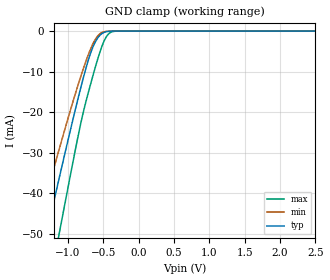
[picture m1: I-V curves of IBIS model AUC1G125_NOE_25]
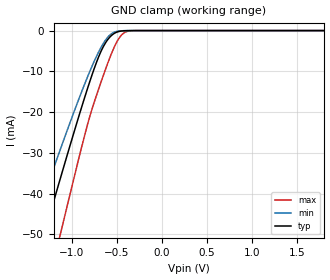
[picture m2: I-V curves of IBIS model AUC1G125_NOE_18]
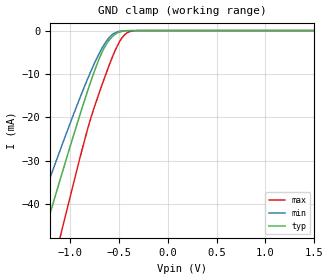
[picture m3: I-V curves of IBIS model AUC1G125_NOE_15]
| TEXAS INSTRUMENTS INCORPORATED
| Standard Linear and Logic Group
| IBIS Model of SN74AUC1G125
| Single Bus Buffer Gate with 3-State Output
| This file contains package information for the following:
|  SOT 5-pin (DBV) package as [Component] AUC1G125_DBV
|  SOT 5-pin (DCK) package as [Component] AUC1G125_DCK
|  DSBGA 5-pin (YEA) package as [Component] AUC1G125_YEA
|  DSBGA 5-pin (YZA) package as [Component] AUC1G125_YZA
|  DSBGA 5-pin (YEP) package as [Component] AUC1G125_YEP
|  DSBGA 5-pin (YZP) package as [Component] AUC1G125_YZP
| This device can be powered at the following Vccs:
|  2.5 volt Vcc
|  1.8 volt Vcc
|  1.5 volt Vcc
|  1.2 volt Vcc
|  0.8 volt Vcc
| This file provides unique models under the [Model Selector] for each Vcc.
| For operation at a specific Vcc, select the appropriate model after each
| [Model Selector] keyword.
[IBIS Ver]   3.2
[Comment char]  |_char
[File Name]   sn74auc1g125.ibs
[File Rev]   1.3 | x_die
[Date]   July 27, 2004
[Source]   Data created from TI-SPICE simulations at TI-SLL.
[Notes]   The following is an IBIS list for the SN74AUC1G125.
   Please contact sllibis@ti.com with questions and
   comments concerning SLL IBIS models.
   - FILE REV HISTORY
   - 1.3 YEP and YZP packages added on 07/27/04
   - The SN74AUC1G125 has output feedback control circuitry.
   This will cause some non-monotonicity warnings.
   - The SN74AUC1G125 inputs has no power clamp diode.
   Therefore, the input power clamp data are not included.
   - The SN74AUC1G125 outputs has no power clamp diode.
   Therefore, the output power clamp data are not included.
   - End point warning due to AC and DC mismatch.
[Disclaimer] Property of Texas Instruments Incorporated.  Unauthorized
   reproduction and/or distribution is strictly prohibited.
   This product is protected under copyright law.
   Created  2002, (C) Copyright  2002, Texas Instruments
   Incorporated, All Rights Reserved
   UNLESS THERE IS A SIGNED, WRITTEN AGREEMENT TO THE
   CONTRARY, TEXAS INSTRUMENTS (TI) IS PROVIDING THE IBIS
   MODELS  AND WITHOUT ANY WARRANTY, EXPRESSED OR
   IMPLIED.  TI assumes no liability for:
   1) the accuracy of the IBIS models provided to your
   company;
   2) the proper functioning of these IBIS Models in your
   design or for any resulting applications; or
   3) infringement of patents, copyrights or intellectual
   property rights resulting from your use of these IBIS
   models.
   TI provides IBIS Models as a service to our customers.
   You and your company shall not distribute, sell or give
   these models to anyone else without prior written
   permission from TI.
   TI reserves the right to make changes to our products or
   to discontinue any semiconductor product or service
   without notice, and advises our customers to obtain the
   latest version of relevant information to verify, before
   placing orders, that the information being relied on is
   current.
   Please be aware that your receipt and use of the IBIS
   information provided shall serve as acceptance of these
   terms and conditions.  If you do not accept these terms,
   you should return or destroy the IBIS models and any
   other accompanying information immediately.
| Component AUC1G125_DBV 5-pin SOT
[Component]   AUC1G125_DBV
[Manufacturer]   Texas Instruments, Inc.
[Package]
|   typ   min   max
R_pkg   2.500e-02   2.100e-02   2.900e-02
L_pkg   1.529e-09   1.312e-09   1.906e-09
C_pkg   1.560e-13   1.100e-13   2.400e-13
[Pin]   signal_name   model_name   R_pin   L_pin   C_pin
1   NOE   AUC1G125_NOE   2.100e-02   1.511e-09   1.440e-13
2   A   AUC1G125_IN   2.300e-02   1.312e-09   1.380e-13
3   GND   GND   2.900e-02   1.906e-09   2.400e-13
4   Y   AUC1G125_OUT   2.600e-02   1.541e-09   1.500e-13
5   VCC   POWER   2.500e-02   1.374e-09   1.100e-13
| Component AUC1G125_DCK 5-pin SOT
[Component]   AUC1G125_DCK
[Manufacturer]   Texas Instruments, Inc.
[Package]
|   typ   min   max
R_pkg   2.000e-02   1.700e-02   2.500e-02
L_pkg   9.980e-10   8.810e-10   1.069e-09
C_pkg   1.460e-13   1.180e-13   2.050e-13
[Pin]   signal_name   model_name   R_pin   L_pin   C_pin
1   NOE   AUC1G125_NOE   1.900e-02   1.069e-09   1.620e-13
2   A   AUC1G125_IN   1.800e-02   8.810e-10   1.210e-13
3   GND   GND   1.700e-02   1.031e-09   2.050e-13
4   Y   AUC1G125_OUT   2.000e-02   9.600e-10   1.240e-13
5   VCC   POWER   2.500e-02   1.049e-09   1.180e-13
| Component AUC1G125_YEA 5-pin NanoStar WCSP
[Component]   AUC1G125_YEA
[Manufacturer]   Texas Instruments, Inc.
[Package]
|   typ   min   max
R_pkg   0.001   0.001   0.001
L_pkg   0.021nH   0.021nH   0.021nH
C_pkg   0.046pF   0.045pF   0.047pF
[Pin]   signal_name   model_name   R_pin   L_pin   C_pin
1   NOE   AUC1G125_NOE   0.001   0.021nH   0.046pF
2   A   AUC1G125_IN   0.001   0.021nH   0.047pF
3   GND   GND   0.001   0.021nH   0.046pF
4   Y   AUC1G125_OUT   0.001   0.021nH   0.045pF
5   VCC   POWER   0.001   0.021nH   0.045pF
| Component AUC1G125_YZA 5-pin NanoFree WCSP
[Component]   AUC1G125_YZA
[Manufacturer]   Texas Instruments, Inc.
[Package]
|   typ   min   max
R_pkg   0.001   0.001   0.001
L_pkg   0.021nH   0.021nH   0.021nH
C_pkg   0.046pF   0.045pF   0.047pF
[Pin]   signal_name   model_name   R_pin   L_pin   C_pin
1   NOE   AUC1G125_NOE   0.001   0.021nH   0.046pF
2   A   AUC1G125_IN   0.001   0.021nH   0.047pF
3   GND   GND   0.001   0.021nH   0.046pF
4   Y   AUC1G125_OUT   0.001   0.021nH   0.045pF
5   VCC   POWER   0.001   0.021nH   0.045pF
| Component AUC1G125_YEP 5-pin DSBGA
[Component]   AUC1G125_YEP
[Manufacturer]   Texas Instruments, Inc.
[Package]
|   typ   min   max
R_pkg   0.001   0.001   0.001
L_pkg   0.021nH   0.021nH   0.021nH
C_pkg   0.046pF   0.045pF   0.047pF
[Pin]   signal_name   model_name   R_pin   L_pin   C_pin
1   NOE   AUC1G125_NOE   0.001   0.021nH   0.046pF
2   A   AUC1G125_IN   0.001   0.021nH   0.047pF
3   GND   GND   0.001   0.021nH   0.046pF
4   Y   AUC1G125_OUT   0.001   0.021nH   0.045pF
5   VCC   POWER   0.001   0.021nH   0.045pF
| Component AUC1G125_YZP 5-pin DSBGA
[Component]   AUC1G125_YZP
[Manufacturer]   Texas Instruments, Inc.
[Package]
|   typ   min   max
R_pkg   0.001   0.001   0.001
L_pkg   0.021nH   0.021nH   0.021nH
C_pkg   0.046pF   0.045pF   0.047pF
[Pin]   signal_name   model_name   R_pin   L_pin   C_pin
1   NOE   AUC1G125_NOE   0.001   0.021nH   0.046pF
2   A   AUC1G125_IN   0.001   0.021nH   0.047pF
3   GND   GND   0.001   0.021nH   0.046pF
4   Y   AUC1G125_OUT   0.001   0.021nH   0.045pF
5   VCC   POWER   0.001   0.021nH   0.045pF
| Model AUC1G125_NOE
[Model Selector]   AUC1G125_NOE
AUC1G125_NOE_25   2.5 volt Vcc
AUC1G125_NOE_18   1.8 volt Vcc
AUC1G125_NOE_15   1.5 volt Vcc
AUC1G125_NOE_12   1.2 volt Vcc
AUC1G125_NOE_08   0.8 volt Vcc
| Model AUC1G125_IN
[Model Selector]   AUC1G125_IN
AUC1G125_IN_25   2.5 volt Vcc
AUC1G125_IN_18   1.8 volt Vcc
AUC1G125_IN_15   1.5 volt Vcc
AUC1G125_IN_12   1.2 volt Vcc
AUC1G125_IN_08   0.8 volt Vcc
| Model AUC1G125_OUT
[Model Selector]   AUC1G125_OUT
AUC1G125_OUT_25   2.5 volt Vcc
AUC1G125_OUT_18   1.8 volt Vcc
AUC1G125_OUT_15   1.5 volt Vcc
AUC1G125_OUT_12   1.2 volt Vcc
AUC1G125_OUT_08   0.8 volt Vcc
| Models and submodels in the file (15): AUC1G125_NOE_25 (Input), AUC1G125_NOE_18 (Input), AUC1G125_NOE_15 (Input), AUC1G125_NOE_12 (Input), AUC1G125_NOE_08 (Input), AUC1G125_IN_25 (Input), AUC1G125_IN_18 (Input), AUC1G125_IN_15 (Input), AUC1G125_IN_12 (Input), AUC1G125_IN_08 (Input), AUC1G125_OUT_25 (3-state), AUC1G125_OUT_18 (3-state), AUC1G125_OUT_15 (3-state), AUC1G125_OUT_12 (3-state), AUC1G125_OUT_08 (3-state)
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[Model]   AUC1G125_NOE_25
Model_type  Input
Vinl=0.7
Vinh=1.7
| variable   typ   min   max
C_comp   2.23pF   1.82pF   2.71pF
[Temperature Range]   40   100   -40
| Ambient temperature   25   85   -40
[Voltage range]   2.5   2.3   2.7
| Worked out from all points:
|   GND clamp passes 1 mA (typ) near -0.55 V on its own axis
[GND Clamp]
| AUC1G125_NOE_25
|   Voltage   I(typ)   I(min)   I(max)
-3.6V     -230.2mA   -193.8mA   -275.4mA
-1.465V   -62.46mA   -50.68mA   -81.32mA
-1.41V    -58.19mA   -47.14mA   -76.26mA
-1.3V     -49.69mA   -40.13mA   -66.14mA
-1.11V    -35.19mA   -28.25mA   -48.67mA
-845mV    -15.76mA   -12.61mA   -24.92mA
-720mV    -7.623mA   -6.181mA   -15.69mA
-625mV    -3.09mA    -2.403mA   -9.633mA
-515mV    -559.5uA   -308.9uA   -3.552mA
-430mV    -73.2uA    -35.77uA   -776.9uA
-325mV    -3.339uA   -2.035uA   -30.74uA
2.5V      313.9pA    402pA      470.4pA
[Model]   AUC1G125_NOE_18
Model_type  Input
Vinl=0.5775
Vinh=1.2675
| variable   typ   min   max
C_comp   2.20pF   1.84pF   2.76pF
[Temperature Range]   40   100   -40
| Ambient temperature   25   85   -40
[Voltage range]   1.8   1.65   1.95
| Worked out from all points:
|   GND clamp passes 1 mA (typ) near -0.55 V on its own axis
[GND Clamp]
| AUC1G125_NOE_18
|   Voltage   I(typ)   I(min)   I(max)
-3.6V     -230.2mA   -193.8mA   -275.4mA
-1.445V   -60.91mA   -49.39mA   -79.48mA
-1.29V    -48.93mA   -39.5mA    -65.22mA
-1.145V   -37.84mA   -30.41mA   -51.89mA
-1.1V     -34.44mA   -27.64mA   -47.76mA
-830mV    -14.72mA   -11.79mA   -23.67mA
-690mV    -5.96mA    -4.844mA   -13.74mA
-565mV    -1.381mA   -914.2uA   -6.102mA
-490mV    -326uA     -167.9uA   -2.495mA
-425mV    -63.97uA   -31.34uA   -688.8uA
-275mV    -662.6nA   -487.6nA   -4.372uA
1.8V      203.2pA    298.4pA    235.5pA
[Model]   AUC1G125_NOE_15
Model_type  Input
Vinl=0.49
Vinh=1.04
| variable   typ   min   max
C_comp   2.22pF   1.84pF   2.76pF
[Temperature Range]   40   100   -40
| Ambient temperature   25   85   -40
[Voltage range]   1.5   1.4   1.6
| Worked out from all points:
|   GND clamp passes 1 mA (typ) near -0.55 V on its own axis
[GND Clamp]
| AUC1G125_NOE_15A
|   Voltage   I(typ)   I(min)   I(max)
-3.6V     -230.2mA   -193.8mA   -275.4mA
-1.39V    -56.64mA   -45.86mA   -74.42mA
-1.25V    -45.85mA   -36.97mA   -61.54mA
-1.095V   -34.06mA   -27.33mA   -47.3mA
-1.05V    -30.68mA   -24.59mA   -43.18mA
-810mV    -13.36mA   -10.7mA    -22.06mA
-685mV    -5.701mA   -4.633mA   -13.41mA
-565mV    -1.381mA   -914.2uA   -6.102mA
-490mV    -326uA     -167.9uA   -2.495mA
-425mV    -63.97uA   -31.34uA   -688.8uA
-280mV    -781.4nA   -563.5nA   -5.358uA
1.5V      165.9pA    259.7pA    172.1pA
